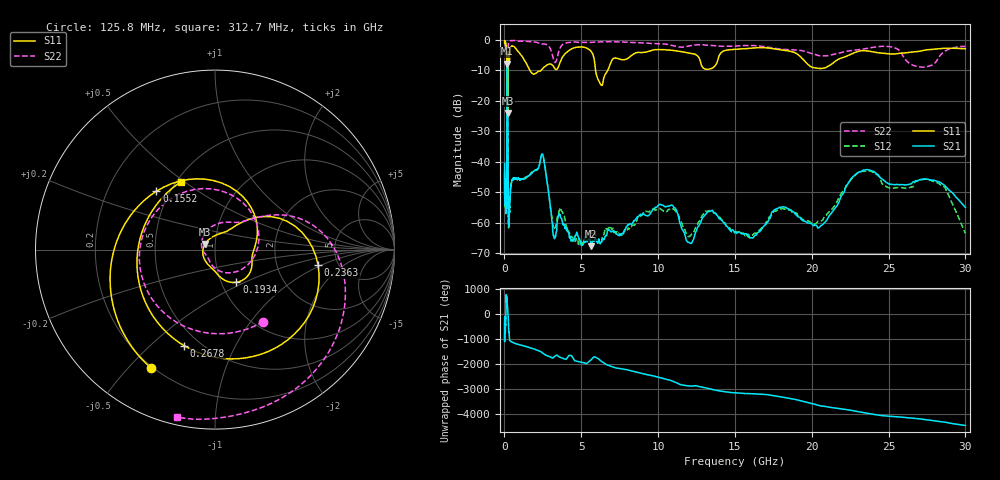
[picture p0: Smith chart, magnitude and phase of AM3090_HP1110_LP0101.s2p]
! Date/Time: Thu, Feb 28, 2019 2:08 PM
! Network Analyzer: Agilent Technologies E8364B Rev: A.07.50.67
! Sweep from 0.010 to 30.000 GHz, 1601 Points, Sweep Type: LOG
! Power Supply: 5.022 V, 0.002 A
# Hz S DB R 50
!freq MagS11 AngS11 MagS21 AngS21 MagS12 AngS12 MagS22 AngS22
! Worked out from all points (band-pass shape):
!   1601 points, 10 MHz to 30 GHz, reference 50 ohm
!   highest |S21| = -7.76 dB at 188.7 MHz (marker M1); lowest = -67.7 dB at 5.64 GHz (marker M2)
!   |S21| within 3 dB of the highest: 171.7 MHz to 210.4 MHz (38.78 MHz wide, 20.3 % of centre)
!   lowest |S11| = -24.0 dB at 209.6 MHz (marker M3), VSWR 1.14, Z = 44.7 + j2.83 ohm
!   |S11| at or under -10 dB: 165.1 MHz to 225.5 MHz (60.4 MHz wide, 30.9 % of centre); 1.657 GHz to 2.378 GHz (721.3 MHz wide, 35.8 % of centre); 5.93 GHz to 6.719 GHz (788.9 MHz wide, 12.5 % of centre)
!   |S22| runs from -24.8 to -0.1 dB; largest |S21 - S12| = 0.012
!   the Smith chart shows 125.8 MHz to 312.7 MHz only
!   S11 on the Smith chart (normalised r, x): 125.8 MHz: 0.19, -0.58; 155.2 MHz: 0.42, +0.35; 193.4 MHz: 1.18, -0.45; 236.3 MHz: 3.51, -0.91; 267.8 MHz: 0.41, -0.65; 312.7 MHz: 0.53, +0.49
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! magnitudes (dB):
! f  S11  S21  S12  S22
! 10 MHz  -0.3  -40.6  -44.8  -0.6
! 38.04 MHz  -0.3  -52.4  -51.2  -1.2
! 125.8 MHz  -2.5  -53.3  -51.6  -6.3
! 144.7 MHz  -4.5  -48.7  -48.5  -7.6
! 155.2 MHz  -6.7  -31.1  -30.9  -9.6
! 188.7 MHz  -12.6  -7.8  -7.8  -22.6
! 193.4 MHz  -13.2  -7.9  -7.9  -20.1
! 209.6 MHz  -24.0  -10.4  -10.4  -13.7
! 236.3 MHz  -4.7  -41.7  -40.8  -2.5
! 267.8 MHz  -5.0  -60.0  -60.9  -0.8
! 312.7 MHz  -7.5  -57.6  -56.6  -0.4
! 550.5 MHz  -2.1  -45.4  -45.8  -0.2
! 2.084 GHz  -10.8  -42.5  -42.6  -0.8
! 2.533 GHz  -9.1  -38.4  -38.4  -1.3
! 3.253 GHz  -9.2  -65.2  -61.8  -7.2
! 5.64 GHz  -3.7  -67.7  -63.4  -0.8
! 6.234 GHz  -14.3  -66.9  -65.5  -0.6
! 7.926 GHz  -6.3  -61.4  -61.9  -0.7
! 20.2 GHz  -9.2  -60.8  -60.4  -4.7
! 23.48 GHz  -3.5  -42.7  -43.1  -2.9
! 27.83 GHz  -3.1  -46.0  -46.3  -8.2
! 30 GHz  -2.9  -55.0  -63.5  -2.1
